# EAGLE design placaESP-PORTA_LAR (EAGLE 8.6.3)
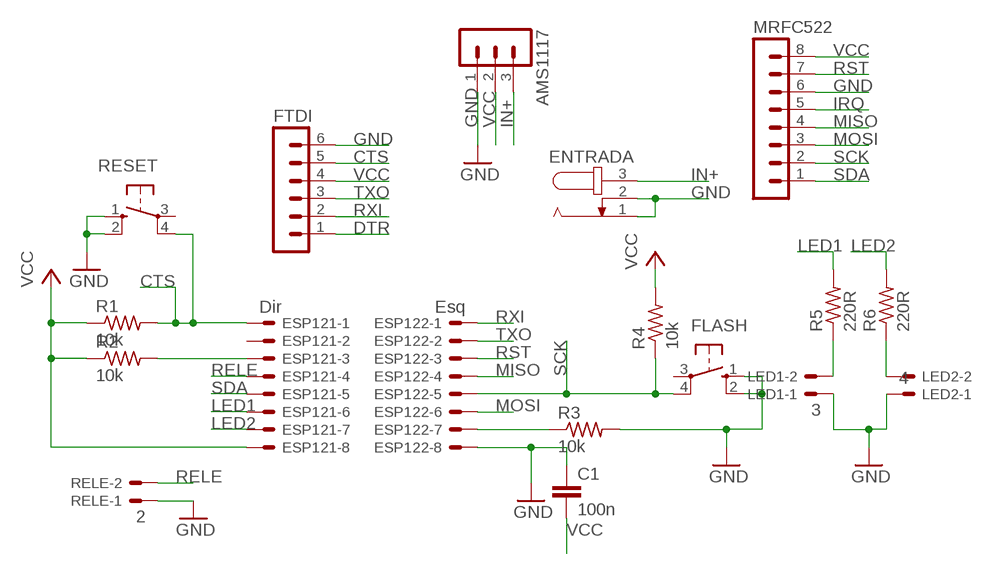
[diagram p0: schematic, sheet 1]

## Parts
AMS1117  MA03-1  [MA03-1]
C1  100n  C-EU025-025X050  [C025-025X050]
ENTRADA  JACK-PLUG0  [SPC4077]
ESP121  Dir  22-23-2081  [22-23-2081]
ESP122  Esq  22-23-2081  [22-23-2081]
FLASH  10-XX  [B3F-10XX]
FTDI  MA06-1  [MA06-1]
LED1  3  22-23-2021  [22-23-2021]
LED2  4  22-23-2021  [22-23-2021]
MRFC522  MA08-1  [MA08-1]
R1  10k  R-US_0207/10  [0207/10]
R2  10k  R-US_0207/10  [0207/10]
R3  10k  R-US_0207/10  [0207/10]
R4  10k  R-US_0207/10  [0207/10]
R5  220R  R-US_0207/10  [0207/10]
R6  220R  R-US_0207/10  [0207/10]
RELE  2  22-23-2021  [22-23-2021]
RESET  10-XX  [B3F-10XX]

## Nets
CTS: ESP121.1 FTDI.5 R1.2 RESET.4(P1)
DTR: FTDI.1
GND: AMS1117.1 C1.1 ENTRADA.1 ENTRADA.2 ESP122.8 FLASH.1(S) FLASH.2(S1) FTDI.6 LED1.1 LED2.1 MRFC522.6 R3.2 RELE.1 RESET.1(S) RESET.2(S1)
IN+: AMS1117.3 ENTRADA.3
IRQ: MRFC522.5
LED1: ESP121.6 R5.2
LED2: ESP121.7 R6.2
MISO: ESP122.4 MRFC522.4
MOSI: ESP122.6 MRFC522.3
N$1: ESP122.7 R3.1
N$2: LED2.2 R6.1
N$3: ESP121.3 R2.2
N$5: LED1.2 R5.1
RELE: ESP121.4 RELE.2
RST: ESP122.3 MRFC522.7
RXI: ESP122.1 FTDI.2
SCK: ESP122.5 FLASH.4(P1) MRFC522.2 R4.1
SDA: ESP121.5 MRFC522.1
TXO: ESP122.2 FTDI.3
VCC: AMS1117.2 C1.2 ESP121.8 FTDI.4 MRFC522.8 R1.1 R2.1 R4.2
Unconnected: ESP121.2 FLASH.3(P) RESET.3(P)

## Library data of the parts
AMS1117 = con-lstb:MA03-1: PIN HEADER; OC_FARNELL: unknown; OC_NEWARK: unknown
C1 = rcl:C-EU: CAPACITOR, European symbol
ENTRADA = con-jack:JACK-PLUG: DC POWER JACK Power Jack, DC, Right Angle, Through Hole, Rated 5A at 16VDC, PC Terminals Distributor: Farnell (www.Farnell.de) Drawing: 84N1161.pdf / 84N1162.pdf Manufacturer: SPC Technology (www.spctechnology.com) Type: SPC4077 / SPC 4078; OC_FARNELL: unknown; OC_NEWARK: unknown
ESP121 ESP122 = con-molex:22-23-2081: .100" (2.54mm) Center Header - 8 Pin; MF: MOLEX; MPN: 22-23-2081; OC_FARNELL: 1756826; OC_NEWARK: 01C7592
FLASH RESET = switch-omron:10-XX: OMRON SWITCH; MPN: B3F-1000; OC_FARNELL: 176432; OC_NEWARK: 36M3542
FTDI = con-lstb:MA06-1: PIN HEADER; OC_FARNELL: unknown; OC_NEWARK: unknown
LED1 LED2 RELE = con-molex:22-23-2021: .100" (2.54mm) Center Header - 2 Pin; MF: MOLEX; MPN: 22-23-2021; OC_FARNELL: 1462926; OC_NEWARK: 25C3832
MRFC522 = con-lstb:MA08-1: PIN HEADER; OC_FARNELL: unknown; OC_NEWARK: unknown
R1-R6 = resistor:R-US_: RESISTOR, American symbol

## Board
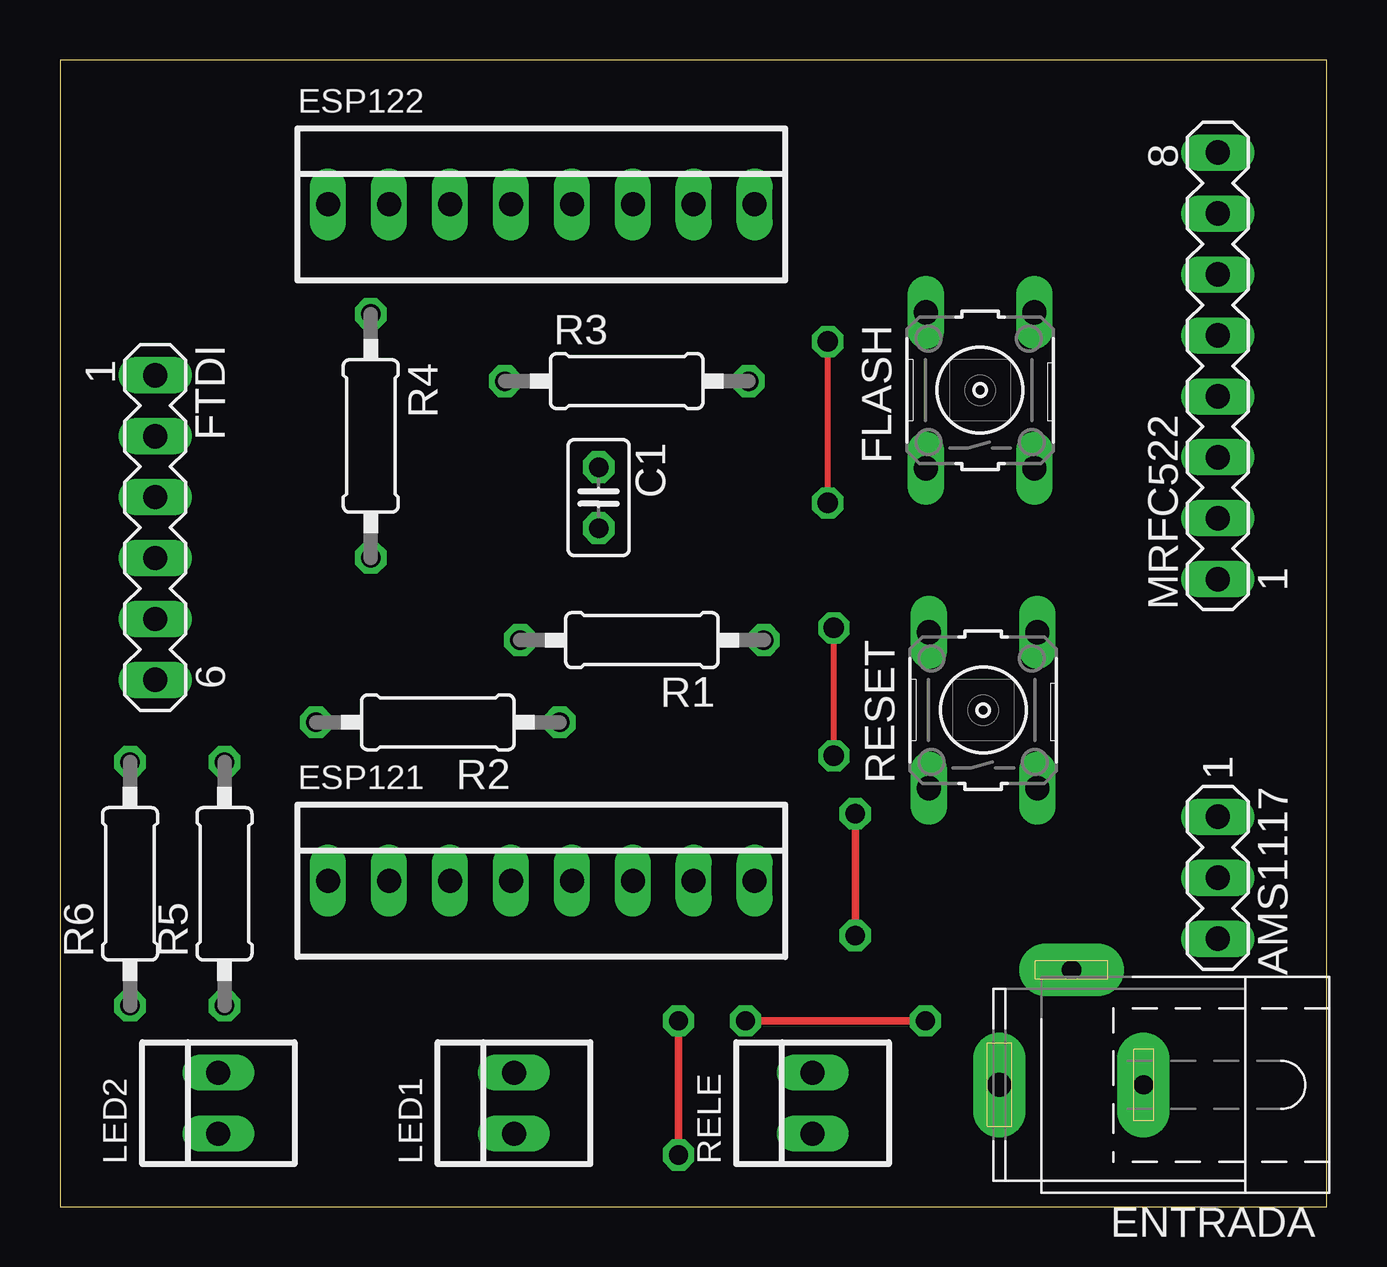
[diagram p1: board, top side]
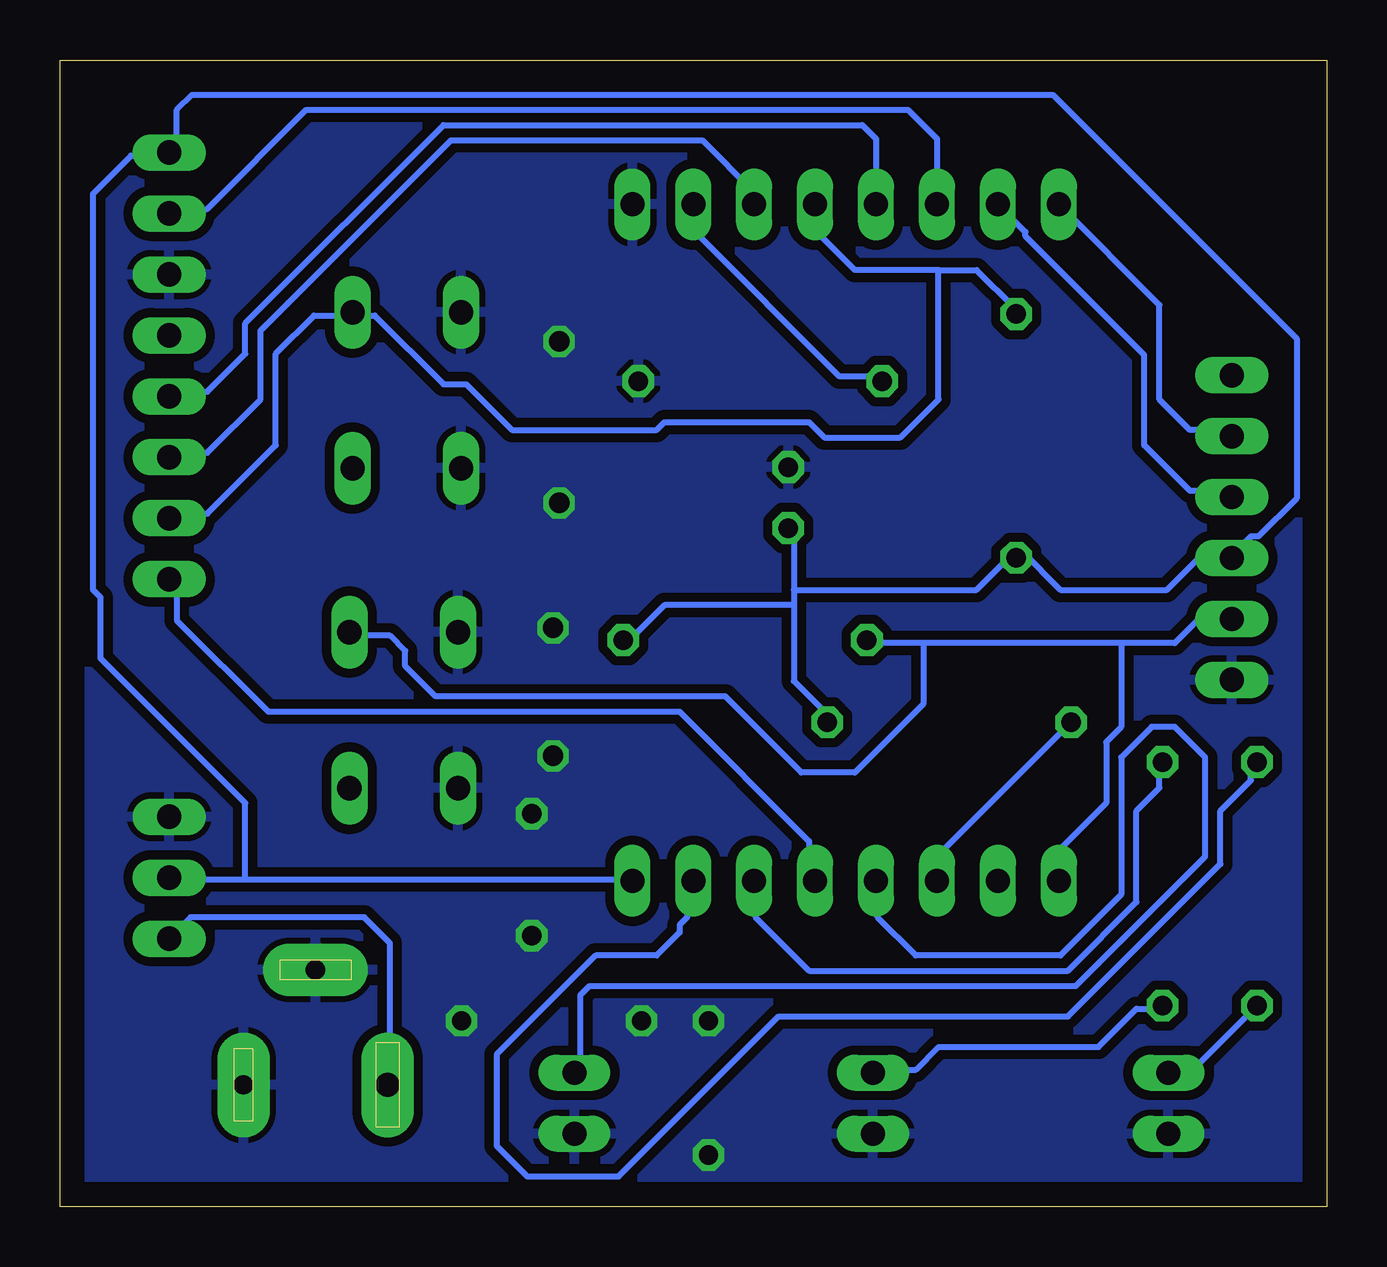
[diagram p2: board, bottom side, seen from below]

Size 52.81 x 47.8 mm. Coordinates in mm from the lower left corner, seen from the top.
Outline: 0,0 52.81,0 52.81,47.8 0,47.8 0,0
Copper layers (1*16): Top 0.035mm / dielectric 1.5mm / Bottom 0.035mm
Design rules "default *": minimum track width 10mil, minimum drill 24mil, track to track 15mil, track to pad 20mil, pad to pad 15mil, via to via 15mil, smd to smd 8mil, copper to edge 40mil, drill to drill 8mil, minimum pad ring 10mil, minimum via ring 8mil, stop-mask expansion 4mil, vias tented up to drill 0mil, thermal gap 10mil

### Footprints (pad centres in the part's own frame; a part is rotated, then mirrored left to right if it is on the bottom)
MA03-1 = drill 1.016 long: 1 -2.54,0; 2 0,0; 3 2.54,0
C025-025X050 = drill 0.813 octagon: 1 -1.27,0; 2 1.27,0
SPC4077 = drill 0.8 pad 2.184 long: 1 -3,0; 2 0,-4.8 | drill 1 pad 2.184 long: 3 3,0
22-23-2081 = drill 1 long: 1 -8.89,0; 2 -6.35,0; 3 -3.81,0; 4 -1.27,0; 5 1.27,0; 6 3.81,0; 7 6.35,0; 8 8.89,0
B3F-10XX = drill 1.016 long: 1 -3.251,2.261; 2 3.251,2.261; 3 -3.251,-2.261; 4 3.251,-2.261
MA06-1 = drill 1.016 long: 1 -6.35,0; 2 -3.81,0; 3 -1.27,0; 4 1.27,0; 5 3.81,0; 6 6.35,0
22-23-2021 = drill 1 long: 1 -1.27,0; 2 1.27,0
MA08-1 = drill 1.016 long: 1 -8.89,0; 2 -6.35,0; 3 -3.81,0; 4 -1.27,0; 5 1.27,0; 6 3.81,0; 7 6.35,0; 8 8.89,0
0207/10 = drill 0.813 octagon: 1 -5.08,0; 2 5.08,0

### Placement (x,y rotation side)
AMS1117  48.26,13.72 270 top
C1  22.45,29.56 270 top
ENTRADA  42.16,5.08 180 top
ESP121  20.07,13.59 0 top
ESP122  20.07,41.78 0 top
FLASH  38.35,34.04 90 top
FTDI  3.97,28.31 270 top
LED1  18.92,4.32 90 top
LED2  6.6,4.32 90 top
MRFC522  48.26,35.05 90 top
R1  24.26,23.62 180 top
R2  15.75,20.19 180 top
R3  23.62,34.42 0 top
R4  12.95,32.13 270 top
R5  6.86,13.46 90 top
R6  2.92,13.46 90 top
RELE  31.37,4.32 90 top
RESET  38.48,20.7 90 top

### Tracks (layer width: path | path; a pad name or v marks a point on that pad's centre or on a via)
CTS
  Bottom 0.254: 8.57,23.5 6.35,23.5 5.4,24.45 4.13,24.45 FTDI.5 | 8.57,23.5 16.83,23.5 | 16.83,23.5 19.05,23.5 R1.2 | 8.57,23.5 8.57,20 9.21,19.37 9.21,16.83 11.11,14.92 11.11,13.65 ESP121.1 | 16.83,23.5 16.83,20.95 19.68,18.1 21.91,18.1 25.08,21.27 37.15,21.27 38.42,22.54 38.42,23.18 39.05,23.81 40.64,23.81 RESET.4
GND  (via drill 0.8 pad 1.3, 0.85 pad 1.3)
  Top 0.254: v32.26,18.8 v32.26,24.13 | v32,29.34 v32,36.07
  Top 0.305: v33.15,16.38 v33.15,11.3 | v25.78,2.16 v25.78,7.75 | v28.57,7.75 v36.07,7.75
  pour Bottom: 0,0 53.35,0 53.35,48.76 0,48.76
IN+
  Bottom 0.254: 48.26,11.11 AMS1117.3 47.37,12.06 40.13,12.06 39.06,11 39.06,5.18 ENTRADA.3
LED1
  Bottom 0.254: R5.2 6.99,18.41 6.99,17.46 7.94,16.51 7.94,12.7 10.79,9.84 21.59,9.84 23.81,12.06 23.81,13.34 ESP121.6
LED2
  Bottom 0.254: R6.2 3.17,18.41 3.17,17.78 4.45,16.51 4.45,14.29 10.79,7.94 22.86,7.94 29.53,1.27 33.34,1.27 34.61,2.54 34.61,6.35 30.48,10.48 27.94,10.48 26.99,11.43 26.99,11.75 26.67,12.06 26.67,13.34 ESP121.7
MISO
  Bottom 0.254: MRFC522.4 48.26,33.97 46.67,33.97 45.09,35.56 45.09,36.83 36.83,45.09 19.37,45.09 18.8,44.51 ESP122.4
MOSI
  Bottom 0.254: MRFC522.3 48.26,31.43 46.67,31.43 44.45,33.66 44.45,36.51 36.51,44.45 26.04,44.45 23.88,42.29 ESP122.6
N$1
  Bottom 0.254: R3.1 18.73,34.61 20.32,34.61 26.42,40.7 ESP122.7
N$2
  Bottom 0.254: LED2.2 5.71,5.59 R6.1
N$3
  Bottom 0.254: R2.2 16.26,14.61 ESP121.3
N$5
  Bottom 0.254: R5.1 6.99,8.26 7.94,8.26 9.53,6.67 16.19,6.67 17.14,5.71 18.73,5.71 LED1.2
RELE
  Bottom 0.254: ESP121.4 18.73,13.34 18.73,12.06 17.14,10.48 11.11,10.48 8.57,13.02 8.57,18.73 7.3,20 6.35,20 5.08,18.73 5.08,14.61 10.48,9.21 30.73,9.21 31.11,8.83 31.11,5.71 RELE.2
RST
  Bottom 0.254: MRFC522.7 48.26,41.59 46.67,41.59 42.55,45.72 17.46,45.72 16.26,44.51 ESP122.3
RXI
  Bottom 0.254: FTDI.2 4.13,32.38 5.71,32.38 6.99,33.66 6.99,37.59 ESP122.1
SCK
  Bottom 0.254: 16.19,39.05 19.68,39.05 21.34,40.7 ESP122.5 | 16.19,39.05 14.61,39.05 13.02,37.47 R4.1 | MRFC522.2 48.26,28.89 46.67,28.89 43.81,31.75 43.81,35.56 42.23,37.15 40.64,37.15 FLASH.4 40.32,37.15 39.69,37.15 36.83,34.29 35.88,34.29 33.97,32.38 27.94,32.38 27.62,32.7 21.59,32.7 20.95,32.07 17.78,32.07 16.19,33.66 16.19,39.05
SDA
  Bottom 0.254: ESP121.5 21.59,13.65 21.59,15.24 26.99,20.64 44.13,20.64 47.94,24.45 47.94,25.72 48.26,26.04 MRFC522.1
TXO
  Bottom 0.254: ESP122.2 12.56,40.63 12.56,40.45 7.62,35.51 7.62,31.75 5.71,29.84 4.23,29.84 FTDI.3
VCC
  Bottom 0.254: 22.23,25.72 22.23,28.26 C1.2 | 22.23,25.72 22.23,25.08 | 22.23,25.08 22.23,21.91 20.95,20.64 20.95,20.32 R2.1 | 22.23,25.08 27.62,25.08 28.89,23.81 29.21,23.81 R1.1 | 22.23,25.72 14.61,25.72 13.34,26.99 13.02,26.99 R4.2 12.7,27.3 11.11,25.72 6.67,25.72 5.4,26.99 4.13,26.99 FTDI.4 3.81,27.3 3.17,27.94 2.86,27.94 1.27,29.53 1.27,36.2 11.43,46.35 47.31,46.35 47.94,45.72 47.94,44.45 48.26,44.13 MRFC522.8 48.26,43.81 49.85,43.81 51.44,42.23 51.44,25.72 51.12,25.4 51.12,22.86 45.09,16.83 45.09,13.65 | 45.09,13.65 48.26,13.65 AMS1117.2 | 45.09,13.65 29.21,13.65 ESP121.8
